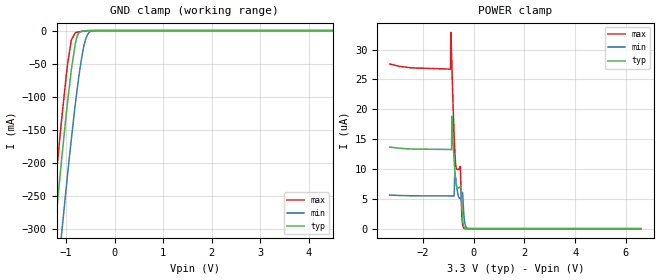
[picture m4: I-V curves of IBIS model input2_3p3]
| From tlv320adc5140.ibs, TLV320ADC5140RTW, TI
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|   input2_3p3 Model
[Model]   input2_3p3
Model_type   Input
Vinl = 0.8
Vinh = 2
|   typ   min   max
C_comp   0.8311pF   0.8010pF   0.8702pF
| Where Nom  PVT is Nominal Process, 3.3V, 27C
|   Fast PVT is Strong Process,  3.6V, -40C
|   Slow PVT is Weak Process,   3.0V, 150C
[Voltage Range]   3.3   3   3.6
|Junction Temperature
[Temperature Range]   27   150   -40
[Power Clamp Reference]   3.3   3   3.6
[GND Clamp Reference]   0   0   0
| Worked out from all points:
|   GND clamp passes 1 mA (typ) near -0.68 V on its own axis
[GND Clamp]
|   Voltage   I(typ)   I(min)   I(max)
-3.3V     -2.018A    -2.043A    -2.005A
-1.31V    -362.7mA   -474mA     -303.1mA
-1.261V   -323.1mA   -434.9mA   -263.2mA
-1.211V   -284mA     -396.1mA   -223.8mA
-1.092V   -193mA     -305.2mA   -132.8mA
-963.6mV  -101.9mA   -211.4mA   -46.18mA
-894.3mV  -58.93mA   -163.7mA   -14.07mA
-815.1mV  -20.58mA   -112.8mA   -3.323mA
-745.8mV  -4.334mA   -72.66mA   -2.123mA
-636.9mV  -521.9uA   -23.74mA   -725uA
-468.6mV  -10.75uA   -628.3uA   -11.46uA
6.6V      0A         0A         0A
[POWER Clamp]
|   Voltage   I(typ)   I(min)   I(max)
-3.3V     13.66uA    5.637uA    27.59uA
-904.2mV  13.27uA    5.479uA    26.74uA
-894.3mV  13.27uA    5.479uA    32.89uA
-864.6mV  13.21uA    5.479uA    29.23uA
-854.7mV  18.85uA    5.479uA    27.68uA
-765.6mV  11.55uA    5.465uA    15.82uA
-716.1mV  8.649uA    8.83uA     11.48uA
-518.1mV  7.025uA    5.048uA    10.44uA
-458.7mV  3.499uA    5.551uA    2.172uA
-379.5mV  267.3nA    2.28uA     60.03nA
-231mV    0A         34.8nA     0A
6.6V      0A         0A         0A
